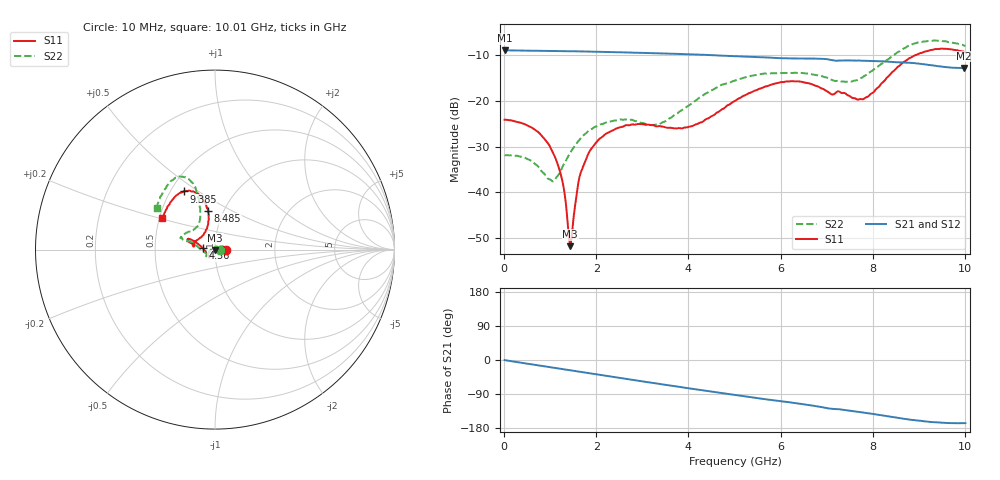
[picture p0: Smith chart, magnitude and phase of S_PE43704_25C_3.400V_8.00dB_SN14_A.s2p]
! Device ID: PE43704
! Dir: z:\PE43704\PE43704_Char_1_20130516\PE43704\AMB\3p400V\8p00dB
! Serial: 14
! Insertion: A
! Impedance: 50 ohm
! Temp: Amb
! VDD: 3.400V
! Attenuation Step: 8.00dB
! IDD: 1.140048e-01mA
#  Hz  S  RI  R  50
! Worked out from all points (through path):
!   401 points, 10 MHz to 10.01 GHz, reference 50 ohm
!   highest |S21| = -8.97 dB at 10 MHz (marker M1); lowest = -12.8 dB at 9.985 GHz (marker M2)
!   group delay of S21, straight-line fit = 48.1 ps
!   lowest |S11| = -51.8 dB at 1.435 GHz (marker M3), VSWR 1.01, Z = 50.2 - j0.192 ohm
!   |S11| at or under -10 dB: start of sweep to 8.935 GHz
!   |S22| runs from -37.6 to -6.8 dB; largest |S21 - S12| = 0.0027
!   S11 on the Smith chart (normalised r, x): 10 MHz: 1.13, +0.00; 4.56 GHz: 0.87, +0.02; 8.485 GHz: 0.85, +0.38; 9.385 GHz: 0.58, +0.44; 10.01 GHz: 0.52, +0.21
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1e7  0.062 0.000177  0.3562 -0.00127  0.3563 -0.00128  0.0253 0.000244
5.35e8  0.0506 0.0158  0.3476 -0.0638  0.3475 -0.0636  0.0163 0.0159
9.85e8  0.0285 0.0152  0.3322 -0.1138  0.3321 -0.1137  -0.00314 0.0135
1.235e9  0.0136 0.00701  0.3202 -0.1407  0.3202 -0.1404  -0.0168 0.00485
1.435e9  0.00173 -0.00191  0.309 -0.1606  0.3089 -0.1604  -0.0268 -0.0048
1.485e9  -0.000898 -0.00404  0.3061 -0.1654  0.3061 -0.1654  -0.0288 -0.00735
1.61e9  -0.00838 -0.00959  0.2983 -0.1775  0.2982 -0.1773  -0.0334 -0.014
1.685e9  -0.011 -0.0137  0.2933 -0.1845  0.2933 -0.1844  -0.0364 -0.0177
1.885e9  -0.0191 -0.0226  0.2791 -0.2021  0.2792 -0.202  -0.0404 -0.027
2.235e9  -0.0269 -0.0351  0.2522 -0.2303  0.2523 -0.2302  -0.0458 -0.0367
3.36e9  -0.036 -0.0388  0.1501 -0.294  0.1505 -0.2937  -0.052 -0.0194
4.01e9  -0.0498 -0.0149  0.0848 -0.3106  0.0852 -0.3107  -0.0887 0.0088
4.56e9  -0.0695 0.00962  0.0293 -0.313  0.0298 -0.313  -0.128 0.0408
5.01e9  -0.0946 0.0316  -0.0121 -0.3069  -0.0118 -0.3071  -0.16 0.0472
5.96e9  -0.1455 0.0604  -0.0904 -0.2787  -0.0894 -0.2788  -0.1897 0.0647
6.685e9  -0.1456 0.0424  -0.1461 -0.25  -0.1464 -0.2496  -0.1768 0.0821
7.735e9  -0.0714 0.0761  -0.2032 -0.1849  -0.2029 -0.1851  -0.0875 0.1533
8.36e9  -0.0357 0.1864  -0.2285 -0.1375  -0.2276 -0.1388  -0.089 0.2774
8.485e9  -0.0386 0.2152  -0.2327 -0.1261  -0.231 -0.1272  -0.0968 0.3092
9.385e9  -0.1744 0.3238  -0.2315 -0.0637  -0.2323 -0.0632  -0.2284 0.3926
9.985e9  -0.2876 0.1848  -0.2217 -0.0525  -0.2229 -0.0527  -0.3208 0.2397
1.001e10  -0.2925 0.1747  -0.2226 -0.053  -0.2241 -0.0534  -0.3246 0.2322
